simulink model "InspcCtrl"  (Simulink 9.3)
settings: Solver=FixedStepDiscrete  StartTime=0.0  StopTime=100000  FixedStep=Tstep  RelTol=1e-3  EnableMultiTasking=on
PreLoadFcn:
  | InspcCtrl.InspcCtrl_init();
InitFcn:
  | InspcCtrl.InspcCtrl_init();
StartFcn:
  | InspcCtrl.InspcCtrl_init();
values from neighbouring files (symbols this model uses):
  Tinit = 0.001    [InspcCtrl_init.m]    (also in TestOrthOscObjO_init.m = 0.1; TestOrthOsc_init.m; Test_PIDctrl_init.m; Test_LibVishia_Inspc_init.m = 0.002)
  Tstep = 0.0001    [InspcCtrl_init.m]    (also in TestOrthOscObjO_init.m = 0.0005; stimuli_Smlk.m = 0.001; TestOrthOsc_init.m = 5e-05; Test_PIDctrl_init.m)
undefined symbols (not defined in the file or in its folder): intmax, s1, s2, T1, test, TIs, v2, validy
libraries: libVishia_Inspc x36, libVishia_Ctrl x3, libVishia_CtrlSfn x2, libVishia_Conv x2, simulink x1

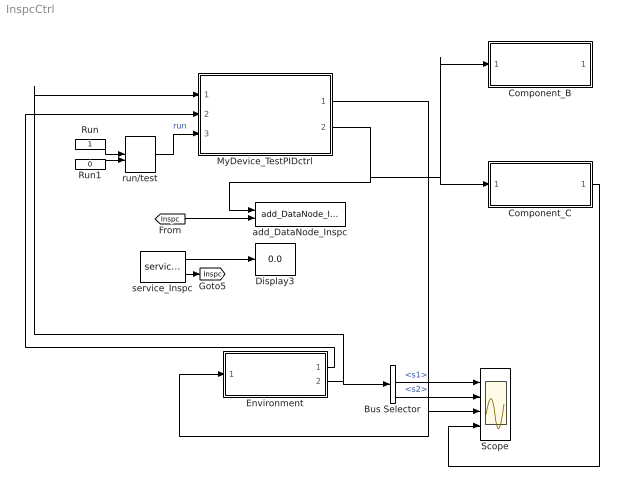
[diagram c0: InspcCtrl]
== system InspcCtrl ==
  Bus Selector : BusSelector  OutputSignals=s1,s2
  Component_B : Subsystem  Commented=on
  Component_C : Subsystem
  Display3 : Display
  Environment : Subsystem
  MyDevice_TestPIDctrl : Subsystem
  Run : Constant  OutDataTypeStr=boolean
  Run1 : Constant  Value=0  OutDataTypeStr=boolean
  Scope : Scope  NumInputPorts=4
  add_DataNode_Inspc : libVishia_Inspc/add_DataNode_Inspc  name1Refl='myDevice'  name2Refl=''
  run/test : ManualSwitch  CurrentSetting=0
  service_Inspc : libVishia_Inspc/service_Inspc  Tstep=Tstep  IpPort='UDP:0.0.0.0:60094'
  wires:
  MyDevice_TestPIDctrl/1(Out1) -> Environment/1(In1), Scope/3
  Environment/2(Out1) -> MyDevice_TestPIDctrl/1(In1), Bus Selector/1
  Bus Selector/1 -> Scope/1  "<s1>"
  service_Inspc/2 -> [Inspc]
  service_Inspc/1 -> Display3/1
  [Inspc] -> add_DataNode_Inspc/2
  MyDevice_TestPIDctrl/2(Out2) -> add_DataNode_Inspc/1, Component_B/1(In1), Component_C/1(In1)
  Bus Selector/2 -> Scope/2  "<s2>"
  Run/1 -> run/test/1
  Run1/1 -> run/test/2
  run/test/1 -> MyDevice_TestPIDctrl/3(In2)  "run"
  Environment/1(Out2) -> MyDevice_TestPIDctrl/2(In3)
  Component_C/1(Out1) -> Scope/4

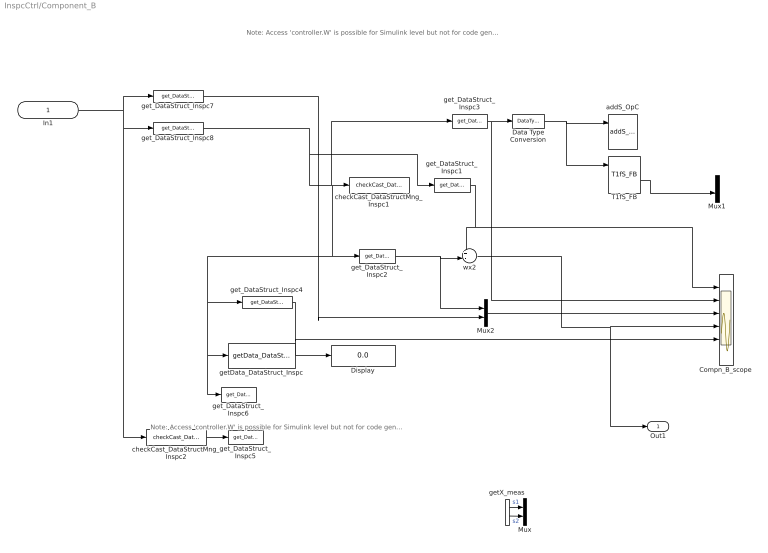
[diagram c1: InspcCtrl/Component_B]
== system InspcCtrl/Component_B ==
  note: Note: Access 'controller.W' is possible for Simulink level but not for code generation. Necessary to create special parameter in runtime. The necessary information for code generation are available only after init_... war run. With String processing in tlc it may be able. But tlc as less features for String processing.
  note: Note: Access 'controller.W' is possible for Simulink level but not for code generation. Necessary to create special parameter in runtime. The necessary information for code generation are available only after init_... war run. With String processing in tlc it may be able. But tlc as less features for String processing.
  In1 : Inport  OutDataTypeStr=uint32  PortDimensions=1  SampleTime=Tinit
  Compn_B_scope : Scope  NumInputPorts=6
  Data Type Conversion : DataTypeConversion  OutDataTypeStr=double
  Display : Display
  Mux : Mux  Commented=on  Inputs=2
  Mux1 : Mux  Inputs=2
  Mux2 : Mux  Inputs=2
  T1fS_FB : libVishia_Ctrl/T1fS_FB  T1=100  P_TA=Tstep
  addS_OpC : libVishia_Ctrl/addS_OpC  init=0  Tstep=-1
  checkCast_DataStructMng_Inspc1 : libVishia_Inspc/checkCast_DataStruct_Inspc  Commented=on  typeData='Controller_B_ObjMod'  headerfile=''
  checkCast_DataStructMng_Inspc2 : libVishia_Inspc/checkCast_DataStruct_Inspc  Commented=on  typeData='Device_ObjMod'  headerfile=''
  getData_DataStruct_Inspc : libVishia_Inspc/getData_DataStruct_Inspc  Commented=on  Tstep=Tstep  show='wxP'  typeName='F: wxP'  typedata=''  datapath='pid2'  header=''
  getX_meas : S-Function  Commented=on  FunctionName=out_MeasPrep_ProgrSimpleExmplA_SfOp  SFunctionDeploymentMode=off  EnableBusSupport=off
  get_DataStruct_Inspc1 : libVishia_Inspc/get_DataStruct_Inspc  show='test'  Tstep=Tstep  name1='F2:test'  headerfile=''
  get_DataStruct_Inspc2 : libVishia_Inspc/get_DataStruct_Inspc  show='xs'  Tstep=Tstep  name1='F2:xs'  headerfile=''
  get_DataStruct_Inspc3 : libVishia_Inspc/get_DataStruct_Inspc  show='yctrl'  Tstep=Tstep  name1='F2:yctrl'  headerfile=''
  get_DataStruct_Inspc4 : libVishia_Inspc/get_DataStruct_Inspc  show='controller.W'  Tstep=Tstep  name1="'F:  pid2.wxP'"  headerfile=''
  get_DataStruct_Inspc5 : libVishia_Inspc/get_DataStruct_Inspc  Commented=on  show='show'  Tstep=Tstep  name1='W'  headerfile=''
  get_DataStruct_Inspc6 : libVishia_Inspc/get_DataStruct_Inspc  Commented=on  show='s'  Tstep=Tstep  name1='s'  headerfile=''
  get_DataStruct_Inspc7 : libVishia_Inspc/get_DataStruct_Inspc  show='controller.W'  Tstep=Tstep  name1="'(Device_ObjMod*) F2:  controller.W'"  headerfile=''
  get_DataStruct_Inspc8 : libVishia_Inspc/get_DataStruct_Inspc  show='controller'  Tstep=Tinit  name1="'(Device_ObjMod*) Controller_ObjMod:  controller'"  headerfile=''
  wx2 : Sum  Inputs=+-|
  Out1 : Outport
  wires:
  In1/1 -> get_DataStruct_Inspc7/1, get_DataStruct_Inspc8/1, checkCast_DataStructMng_Inspc2/1
  get_DataStruct_Inspc1/1 -> wx2/1, Compn_B_scope/1
  Data Type Conversion/1 -> T1fS_FB/1, addS_OpC/1
  T1fS_FB/2 -> Mux1/2
  get_DataStruct_Inspc2/1 -> Mux2/1, wx2/2
  wx2/1 -> Out1/1, Compn_B_scope/4
  get_DataStruct_Inspc3/1 -> Compn_B_scope/2, Data Type Conversion/1
  get_DataStruct_Inspc8/1 -> get_DataStruct_Inspc1/1, checkCast_DataStructMng_Inspc1/1, get_DataStruct_Inspc4/1, getData_DataStruct_Inspc/1, get_DataStruct_Inspc6/1, get_DataStruct_Inspc2/1, get_DataStruct_Inspc3/1
  checkCast_DataStructMng_Inspc2/1 -> get_DataStruct_Inspc5/1
  get_DataStruct_Inspc4/1 -> Compn_B_scope/5, Display/1
  getX_meas/1 -> Mux/1  "s1"
  getX_meas/2 -> Mux/2  "s2"
  Mux/1 -> ?
  Mux2/1 -> Compn_B_scope/3
  get_DataStruct_Inspc7/1 -> Mux2/2

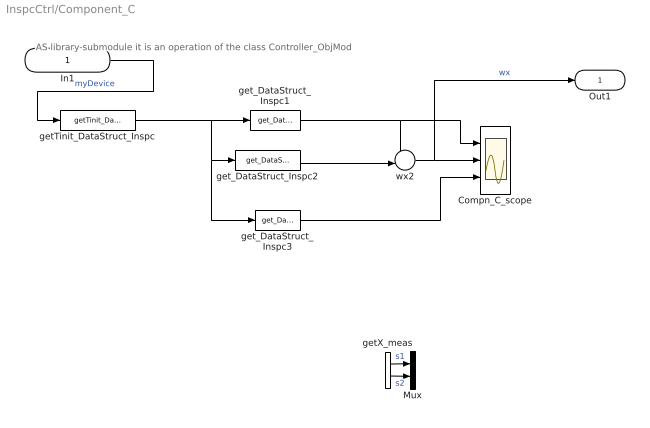
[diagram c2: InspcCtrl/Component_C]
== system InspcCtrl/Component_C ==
  note: AS library-submodule it is an operation of the class Controller_ObjMod
  In1 : Inport  OutDataTypeStr=uint32  PortDimensions=1  SampleTime=Tinit
  Compn_C_scope : Scope  NumInputPorts=3
  Mux : Mux  Commented=on  Inputs=2
  getTinit_DataStruct_Inspc : libVishia_Inspc/getTinit_DataStruct_Inspc  show='=controller'  typeName='(Device_ObjMod) controller: Controller_ObjMod '  headerfile='genSrcInspc/Controller_ObjMod.h'
  getX_meas : S-Function  Commented=on  FunctionName=out_MeasPrep_ProgrSimpleExmplA_SfOp  SFunctionDeploymentMode=off  EnableBusSupport=off
  get_DataStruct_Inspc1 : libVishia_Inspc/get_DataStruct_Inspc  show='W'  Tstep=Tstep  name1='W: F*2'  headerfile=''
  get_DataStruct_Inspc2 : libVishia_Inspc/get_DataStruct_Inspc  show='xs'  Tstep=Tstep  name1='xs: F*2'  headerfile=''
  get_DataStruct_Inspc3 : libVishia_Inspc/get_DataStruct_Inspc  show='yctrl'  Tstep=Tstep  name1='yctrl :F*2'  headerfile=''
  wx2 : Sum  Inputs=+-|
  Out1 : Outport
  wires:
  get_DataStruct_Inspc2/1 -> wx2/2
  getX_meas/1 -> Mux/1  "s1"
  getX_meas/2 -> Mux/2  "s2"
  wx2/1 -> Compn_C_scope/2, Out1/1  "wx"
  get_DataStruct_Inspc3/1 -> Compn_C_scope/3
  getTinit_DataStruct_Inspc/1 -> get_DataStruct_Inspc3/1, get_DataStruct_Inspc2/1, get_DataStruct_Inspc1/1
  In1/1 -> getTinit_DataStruct_Inspc/1  "myDevice"
  get_DataStruct_Inspc1/1 -> wx2/1, Compn_C_scope/1

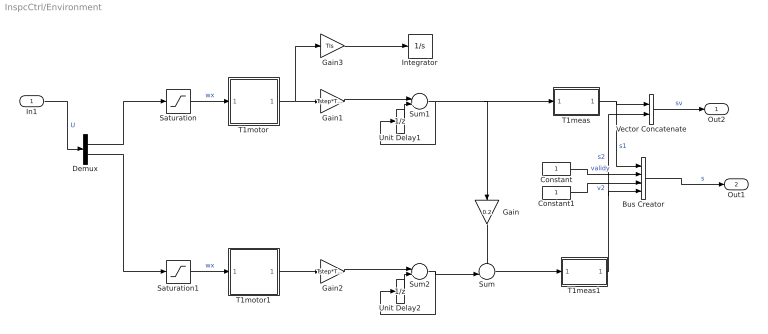
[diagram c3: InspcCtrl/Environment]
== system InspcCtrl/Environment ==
  In1 : Inport  PortDimensions=2
  Bus Creator : BusCreator  Inputs=s1,validy,v2,s2  OutDataTypeStr=Bus: Input_MeasPrep_ProgrSimpleExmplA
  Constant : Constant  OutDataTypeStr=uint16
  Constant1 : Constant  OutDataTypeStr=uint16
  Demux : Demux  Outputs=2
  Gain : Gain  Gain=0.2
  Gain1 : Gain  Gain=Tstep*TIs
  Gain2 : Gain  Gain=Tstep*TIs
  Gain3 : Gain  Commented=on  Gain=TIs
  Integrator : Integrator  Commented=on
  Saturation : Saturate
  Saturation1 : Saturate
  Sum : Sum  Inputs=++|
  Sum1 : Sum  Inputs=|++
  Sum2 : Sum  Inputs=|++
  T1meas : Subsystem
  T1meas1 : Subsystem
  T1motor : Subsystem
  T1motor1 : Subsystem
  Unit Delay1 : UnitDelay  SampleTime=-1  HasFrameUpgradeWarning=on
  Unit Delay2 : UnitDelay  SampleTime=-1  HasFrameUpgradeWarning=on
  Vector Concatenate : Concatenate
  Out2 : Outport  OutDataTypeStr=single
  Out1 : Outport  Port=2  OutDataTypeStr=Bus: Input_MeasPrep_ProgrSimpleExmplA
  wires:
  In1/1 -> Demux/1  "U"
  Saturation/1 -> T1motor/1(In2)  "wx"
  Gain1/1 -> Sum1/1
  T1motor/1(Out2) -> Gain3/1, Gain1/1
  Sum1/1 -> Gain/1, T1meas/1(In2), Unit Delay1/1
  Unit Delay1/1 -> Sum1/2
  Bus Creator/1 -> Out1/1  "s"
  T1meas/1(Out2) -> Vector Concatenate/1, Bus Creator/1  "s1"
  Demux/1 -> Saturation/1
  Demux/2 -> Saturation1/1
  Unit Delay2/1 -> Sum2/2
  T1motor1/1(Out2) -> Gain2/1
  Gain2/1 -> Sum2/1
  Saturation1/1 -> T1motor1/1(In2)  "wx"
  Sum2/1 -> Sum/2, Unit Delay2/1
  Sum/1 -> T1meas1/1(In2)
  Gain/1 -> Sum/1
  T1meas1/1(Out2) -> Vector Concatenate/2, Bus Creator/4  "s2"
  Gain3/1 -> Integrator/1
  Vector Concatenate/1 -> Out2/1  "sv"
  Constant/1 -> Bus Creator/2  "validy"
  Constant1/1 -> Bus Creator/3  "v2"

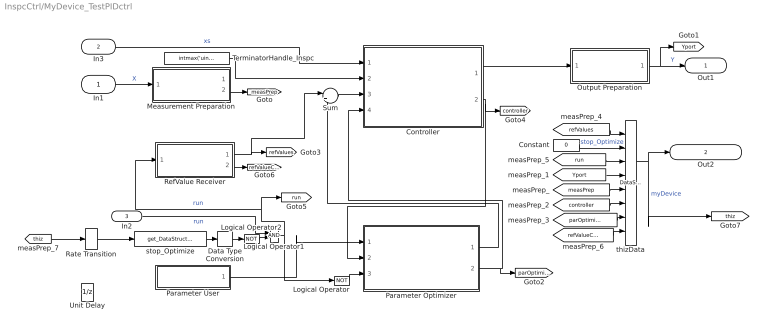
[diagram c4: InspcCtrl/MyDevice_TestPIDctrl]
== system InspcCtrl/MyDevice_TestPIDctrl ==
  In1 : Inport  OutDataTypeStr=Bus: Input_MeasPrep_ProgrSimpleExmplA
  In3 : Inport  Port=2  OutDataTypeStr=single  SampleTime=Tstep
  In2 : Inport  Port=3  OutDataTypeStr=boolean
  Constant : Constant  Value=0  OutDataTypeStr=uint16
  Controller : Subsystem
  Data Type Conversion : DataTypeConversion  OutDataTypeStr=boolean
  Logical Operator : Logic  Operator=NOT  IconShape=distinctive  AllPortsSameDT=off  OutDataTypeStr=boolean
  Logical Operator1 : Logic  IconShape=distinctive  AllPortsSameDT=off  OutDataTypeStr=boolean
  Logical Operator2 : Logic  Operator=NOT  IconShape=distinctive  AllPortsSameDT=off  OutDataTypeStr=boolean
  Measurement Preparation : Subsystem  Commented=on
  Output Preparation : Subsystem
  Parameter Optimizer : Subsystem
  Parameter User : Subsystem
  Rate Transition : RateTransition  OutPortSampleTime=Tstep
  RefValue Receiver : Subsystem
  Sum : Sum  Inputs=|++
  TerminatorHandle_Inspc : Constant  Value=intmax('uint32')  OutDataTypeStr=uint32  SampleTime=Tinit
  Unit Delay : UnitDelay  SampleTime=-1  HasFrameUpgradeWarning=on
  stop_Optimize : libVishia_Inspc/get_DataStruct_Inspc  show='stop_Optimize'  Tstep=Tstep  name1='(Device_ObjMod) stop_Optimize :W'  headerfile=''
  thizData : libVishia_Inspc/DataStructMng_Inspc  dirGenSource=dstPathGenDataStruct  typeData='Device_ObjMod'  inherit=off  chain=off  inputs=|
      | refValues;
      | =stop_Optimize;
      | run;
      | Yport;
      | measPrep :MeasPrep_ProgrSimpleExmplA ;
      | =controller :Controller_ObjMod;
      | =parOptimizer : ParamOptimizer_ObjMod;
      | =refValueCtrl :RefValueCtrl;
  Out1 : Outport  OutDataTypeStr=single  PortDimensions=2
  Out2 : Outport  Port=2  OutDataTypeStr=uint32  PortDimensions=1
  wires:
  RefValue Receiver/1(Out2) -> Sum/1, [refValues]
  Output Preparation/1(Out2) -> [Yport], Out1/1  "Y"
  Controller/1(Out2) -> Output Preparation/1(In3)
  Parameter Optimizer/1(Out1) -> Sum/2
  In1/1 -> Measurement Preparation/1(In1)  "X"
  Parameter User/1(Out2) -> Parameter Optimizer/1(In2)
  Logical Operator/1 -> Parameter Optimizer/3(In1)
  Logical Operator1/1 -> [run], RefValue Receiver/1(In1), Logical Operator/1  "run"
  Sum/1 -> Controller/3(In2)
  In3/1 -> Controller/1(In3)  "xs"
  [Yport] -> thizData/4
  [refValues] -> thizData/1
  Controller/2(Out3) -> Parameter Optimizer/2(In3), [controller]
  Measurement Preparation/2(Out2) -> [measPrep]
  thizData/1 -> [thiz], Out2/1  "myDevice"
  Parameter Optimizer/2(Out3) -> Controller/4(In4), [parOptimizer]
  [run] -> thizData/3
  [measPrep] -> thizData/5
  [controller] -> thizData/6
  [parOptimizer] -> thizData/7
  Constant/1 -> thizData/2  "stop_Optimize"
  RefValue Receiver/2(Out3) -> [refValueCtrl]
  [refValueCtrl] -> thizData/8
  TerminatorHandle_Inspc/1 -> Controller/2(In1)
  In2/1 -> Logical Operator1/1  "run"
  [thiz] -> Rate Transition/1
  Logical Operator2/1 -> Logical Operator1/2
  Data Type Conversion/1 -> Logical Operator2/1
  stop_Optimize/1 -> Data Type Conversion/1
  Rate Transition/1 -> stop_Optimize/1

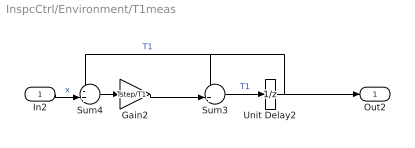
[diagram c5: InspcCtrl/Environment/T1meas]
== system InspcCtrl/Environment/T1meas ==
  In2 : Inport
  Gain2 : Gain  Gain=Tstep/T1
  Sum3 : Sum  Inputs=++|
  Sum4 : Sum  Inputs=-+|
  Unit Delay2 : UnitDelay  SampleTime=-1  HasFrameUpgradeWarning=on
  Out2 : Outport
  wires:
  Sum4/1 -> Gain2/1
  In2/1 -> Sum4/2  "x"
  Sum3/1 -> Unit Delay2/1  "T1"
  Gain2/1 -> Sum3/2
  Unit Delay2/1 -> Sum4/1, Sum3/1, Out2/1  "T1"

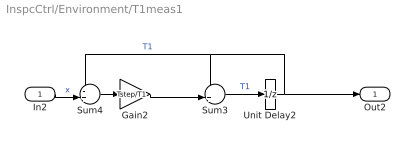
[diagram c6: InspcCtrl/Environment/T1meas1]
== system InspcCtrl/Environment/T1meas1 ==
  In2 : Inport
  Gain2 : Gain  Gain=Tstep/T1
  Sum3 : Sum  Inputs=++|
  Sum4 : Sum  Inputs=-+|
  Unit Delay2 : UnitDelay  SampleTime=-1  HasFrameUpgradeWarning=on
  Out2 : Outport
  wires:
  Sum4/1 -> Gain2/1
  In2/1 -> Sum4/2  "x"
  Sum3/1 -> Unit Delay2/1  "T1"
  Gain2/1 -> Sum3/2
  Unit Delay2/1 -> Sum4/1, Sum3/1, Out2/1  "T1"

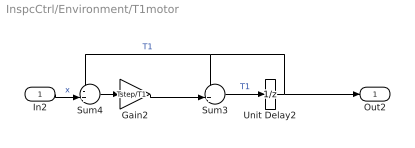
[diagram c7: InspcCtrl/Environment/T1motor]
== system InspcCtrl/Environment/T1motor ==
  In2 : Inport
  Gain2 : Gain  Gain=Tstep/T1
  Sum3 : Sum  Inputs=++|
  Sum4 : Sum  Inputs=-+|
  Unit Delay2 : UnitDelay  SampleTime=-1  HasFrameUpgradeWarning=on
  Out2 : Outport
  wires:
  Sum4/1 -> Gain2/1
  In2/1 -> Sum4/2  "x"
  Sum3/1 -> Unit Delay2/1  "T1"
  Gain2/1 -> Sum3/2
  Unit Delay2/1 -> Sum4/1, Sum3/1, Out2/1  "T1"

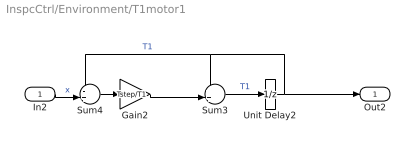
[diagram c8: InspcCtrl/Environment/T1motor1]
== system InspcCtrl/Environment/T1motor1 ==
  In2 : Inport
  Gain2 : Gain  Gain=Tstep/T1
  Sum3 : Sum  Inputs=++|
  Sum4 : Sum  Inputs=-+|
  Unit Delay2 : UnitDelay  SampleTime=-1  HasFrameUpgradeWarning=on
  Out2 : Outport
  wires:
  Sum4/1 -> Gain2/1
  In2/1 -> Sum4/2  "x"
  Sum3/1 -> Unit Delay2/1  "T1"
  Gain2/1 -> Sum3/2
  Unit Delay2/1 -> Sum4/1, Sum3/1, Out2/1  "T1"

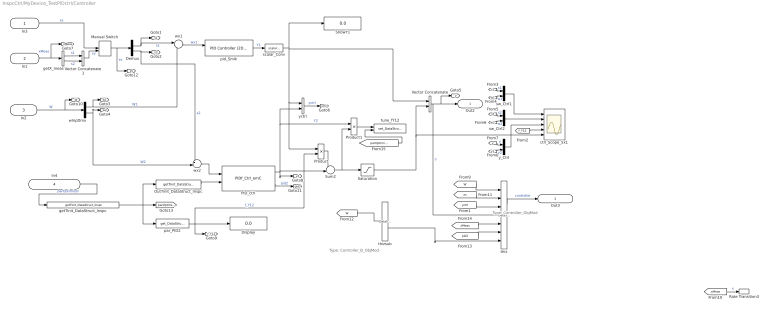
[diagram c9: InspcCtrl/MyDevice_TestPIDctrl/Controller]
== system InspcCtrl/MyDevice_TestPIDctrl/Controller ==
  note: Type: Controller_B_ObjMod
  note: Type: Controller_ObjMod
  In3 : Inport  OutDataTypeStr=single  PortDimensions=2  SampleTime=Tstep
  In1 : Inport  Port=2  OutDataTypeStr=uint32  PortDimensions=1  SampleTime=Tstep
  In2 : Inport  Port=3  OutDataTypeStr=single  PortDimensions=2  SampleTime=Tstep
  In4 : Inport  Port=4  OutDataTypeStr=uint32  PortDimensions=1  SampleTime=Tinit
  Demux : Demux  Outputs=2
  Display : Display
  Manual Switch : ManualSwitch
  OutTinit_DataStruct_Inspc : libVishia_Inspc/getTinit_DataStruct_Inspc  show='par_PID'  typeName='par_PID'  headerfile=''
  PID_ctrl : libVishia_CtrlSfn/PIDf_Ctrl_emC  Tstep=Tstep
  Product : Product
  Product1 : Product
  Rate Transition3 : RateTransition  Commented=on  OutPortSampleTime=Tinit
  Saturation : Saturate  UpperLimit=1  LowerLimit=-1
  ShowY1 : Display
  Sum2 : Sum  Inputs=++|
  Vector Concatenate : Concatenate
  Vector Concatenate1 : Concatenate
  ctrl_Scope_5x1 : Scope  NumInputPorts=5
  getTinit_DataStruct_Inspc : libVishia_Inspc/getTinit_DataStruct_Inspc  show='ParamOptimizer_ObjMod*'  typeName='(ParamOptimizer_ObjMod)'  headerfile=''
  getX_meas : S-Function  Commented=on  FunctionName=out_MeasPrep_ProgrSimpleExmplA_SfOp  SFunctionDeploymentMode=off  EnableBusSupport=off
  par_PID2 : libVishia_Inspc/get_DataStruct_Inspc  show='f_Y12'  Tstep=Tstep  name1='f_Y12 :F'  headerfile=''
  pid_Smlk : simulink/Continuous/PID Controller (2DOF)  Controller=PID  Form=Ideal  TimeDomain=Discrete-time  SampleTime=-1  IntegratorMethod=Backward Euler  FilterMethod=Forward Euler  ControllerParametersSource=internal  P=10  I=5  D=0  UseFilter=on  N=10  b=1  c=1  TunerSelectOption=Transfer Function Based (PID Tuner App)  InitialConditionSource=internal  InitialConditionForIntegrator=0  InitialConditionForFilter=0  DifferentiatorICPrevScaledInput=0  ExternalReset=none  TrackingMode=off  Kt=1  LimitOutput=on  UpperSaturationLimit=1.0  LowerSaturationLimit=-1.0  LinearizeAsGain=off  AntiWindupMode=back-calculation  Kb=1  POutMin=[]  POutMax=[]  IOutMin=[]  IOutMax=[]  DOutMin=[]  DOutMax=[]  NOutMin=[]  NOutMax=[]  bOutMin=[]  bOutMax=[]  cOutMin=[]  cOutMax=[]  SumOutMin=[]  SumOutMax=[]  SaturationOutMin=[]  SaturationOutMax=[]  PParamMin=[]  PParamMax=[]  IParamMin=[]  IParamMax=[]  DParamMin=[]  DParamMax=[]  NParamMin=[]  NParamMax=[]  bParamMin=[]  bParamMax=[]  cParamMin=[]  cParamMax=[]  KbParamMin=[]  KbParamMax=[]  KtParamMin=[]  KtParamMax=[]  KbOutMin=[]  KbOutMax=[]  KtOutMin=[]  KtOutMax=[]  IntegratorOutMin=[]  IntegratorOutMax=[]  FilterOutMin=[]  FilterOutMax=[]  SumI1OutMin=[]  SumI1OutMax=[]  SumI2OutMin=[]  SumI2OutMax=[]  SumI3OutMin=[]  SumI3OutMax=[]  SumI4OutMin=[]  SumI4OutMax=[]  SumDOutMin=[]  SumDOutMax=[]  Sum1OutMin=[]  Sum1OutMax=[]  Sum2OutMin=[]  Sum2OutMax=[]  Sum3OutMin=[]  Sum3OutMax=[]  DifferentiatorOutMin=[]  DifferentiatorOutMax=[]  FilterDiffOutCoefMin=[]  FilterDiffOutCoefMax=[]  ReciprocalOutMin=[]  ReciprocalOutMax=[]  SumDenOutMin=[]  SumDenOutMax=[]  SumNumOutMin=[]  SumNumOutMax=[]  DivideOutMin=[]  DivideOutMax=[]  IntegratorContinuousStateAttributes=''  IntegratorStateMustResolveToSignalObject=off  IntegratorRTWStateStorageClass=Auto  FilterContinuousStateAttributes=''  FilterStateMustResolveToSignalObject=off  FilterRTWStateStorageClass=Auto  ParallelPVariant=Passthrough  IdealPVariant=InternalParameters  IVariant=InternalParameters  DVariant=InternalParameters  bVariant=InternalParameters  cVariant=InternalParameters  IntegratorVariant=Discrete  SatVariant=Enabled  AWVariant=BackCalculation  PCopyVariant=Disabled  TRVariant=Disabled  FdbkBlocksVariant=Feedback  IdealPFdbkVariant=InternalParameters  SatFdbkVariant=Enabled  DerivativeFilterVariant=ForwardEulerFilter  NVariant=InternalParameters  NCopyVariant=Disabled  FilterICVariant=InternalICsFilter  IntegratorICVariant=InternalICs  ExternalResetVariant=Disabled  TRSumVariant=Passthrough  SumFdbkVariant=Enabled  SumVariant=Sum_PID
  scalar_Conv : libVishia_Conv/scalar_Conv  SystemSampleTime=-1
  sw_Ctrl1 : Mux  Inputs=2
  sw_Ctrl2 : Mux  Inputs=2
  thiz : libVishia_Inspc/DataStructMng_Inspc  dirGenSource=dstPathGenDataStruct  typeData='Controller_ObjMod'  inherit=on  chain=off  inputs=|
      | W;
      | xs; //
      | yctrl;
      | Y;
      | =xMeas :MeasPrep_ProgrSimpleExmplA -22;
      | =pid2 : PIDf_Ctrl_emC -22;
  thizsub : libVishia_Inspc/DataStructMng_Inspc  dirGenSource=dstPathGenDataStruct  typeData='Controller_B_ObjMod'  inherit=off  chain=off  inputs=test;
  tune_fY12 : libVishia_Inspc/set_DataStruct_Inspc  show='tune_fY12'  Tstep=Tstep  typeName='(ParamOptimizer_ObjMod) tune_fY12 :F'  headerfile=''
  wInpDmx : Demux  Outputs=2
  wx1 : Sum  Inputs=|-+
  wx2 : Sum  Inputs=-+|
  y_Ctrl : Mux  Inputs=2
  yctrl : Concatenate
  Out2 : Outport  OutDataTypeStr=single  SampleTime=Tstep
  Out3 : Outport  Port=2  OutDataTypeStr=uint32  PortDimensions=1  SampleTime=Tinit
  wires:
  In1/1 -> [xMeas], getX_meas/1  "xMeas"
  pid_Smlk/1 -> scalar_Conv/1  "Y1"
  wInpDmx/1 -> [w1], wx1/2  "W1"
  Demux/2 -> [s2], wx2/1  "s2"
  wx2/1 -> PID_ctrl/1
  Vector Concatenate/1 -> thiz/4, Out2/1, [y]  "Y"
  PID_ctrl/1 -> [y2], Sum2/2, Product1/1, yctrl/2  "Y2"
  sw_Ctrl2/1 -> ctrl_Scope_5x1/2
  PID_ctrl/3 -> [pid2]  "pid2"
  wx1/1 -> pid_Smlk/1  "wx1"
  Demux/1 -> [s1], wx1/1  "s1"
  sw_Ctrl1/1 -> ctrl_Scope_5x1/1
  wInpDmx/2 -> [w2], wx2/2  "W2"
  y_Ctrl/1 -> ctrl_Scope_5x1/3
  Sum2/1 -> Saturation/1, Product1/2
  Product/1 -> Sum2/1
  In2/1 -> [W], wInpDmx/1  "W"
  yctrl/1 -> [yctrl]  "yctrl"
  par_PID2/1 -> Display/1, [f_Y12], Product/2  "f_Y12"
  [s1] -> sw_Ctrl1/1  "s1"
  [w1] -> sw_Ctrl1/2  "w1"
  [w2] -> sw_Ctrl2/2  "w2"
  [s2] -> sw_Ctrl2/1  "s2"
  [y2] -> y_Ctrl/2  "y2"
  [y] -> y_Ctrl/1  "y"
  [xMeas] -> Rate Transition3/1  "x"
  In4/1 -> getTinit_DataStruct_Inspc/1  "parOptimizer"
  [yctrl] -> thiz/3
  [f_Y12] -> ctrl_Scope_5x1/4
  Saturation/1 -> ctrl_Scope_5x1/5, Vector Concatenate/2
  OutTinit_DataStruct_Inspc/1 -> PID_ctrl/2
  Product1/1 -> tune_fY12/1
  [W] -> thiz/1
  thiz/1 -> Out3/1  "controller"
  [W] -> thizsub/1
  [pid2] -> thiz/6
  scalar_Conv/1 -> ShowY1/1, Product/1, yctrl/1, Vector Concatenate/1
  Manual Switch/1 -> [xs], Demux/1  "xs"
  [xs] -> thiz/2
  thizsub/2 -> thiz/7
  getX_meas/1 -> Vector Concatenate1/1  "s1"
  getX_meas/2 -> Vector Concatenate1/2  "s2"
  In3/1 -> Manual Switch/1  "xs"
  Vector Concatenate1/1 -> Manual Switch/2  "sv"
  [xMeas] -> thiz/5
  [parOptimizer] -> tune_fY12/2
  getTinit_DataStruct_Inspc/1 -> par_PID2/1, [parOptimizer], OutTinit_DataStruct_Inspc/1

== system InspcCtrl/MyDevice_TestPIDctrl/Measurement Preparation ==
  In1 : Inport  OutDataTypeStr=Bus: Input_MeasPrep_ProgrSimpleExmplA
  S-Function : S-Function  FunctionName=step_MeasPrep_ProgrSimpleExmplA_SfH  Parameters=Tstep  SFunctionDeploymentMode=off  EnableBusSupport=off
  Out1 : Outport  OutDataTypeStr=uint32
  Out2 : Outport  Port=2  OutDataTypeStr=uint32
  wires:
  In1/1 -> S-Function/1  "X"
  S-Function/2 -> Out2/1  "MeasPrep"
  S-Function/1 -> Out1/1  "Xi"

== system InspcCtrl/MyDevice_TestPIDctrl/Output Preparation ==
  In3 : Inport
  Gain : Gain
  Out2 : Outport
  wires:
  Gain/1 -> Out2/1  "Yport"
  In3/1 -> Gain/1  "Yi"

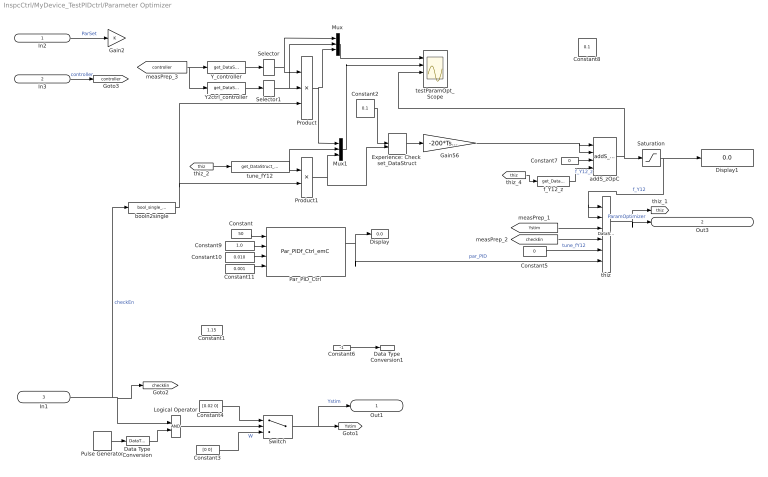
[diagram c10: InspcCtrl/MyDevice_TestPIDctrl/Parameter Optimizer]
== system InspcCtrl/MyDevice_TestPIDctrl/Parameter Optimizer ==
  In2 : Inport  OutDataTypeStr=uint32  PortDimensions=1  SampleTime=Tinit
  In3 : Inport  Port=2  OutDataTypeStr=uint32  PortDimensions=1  SampleTime=Tinit
  In1 : Inport  Port=3  OutDataTypeStr=boolean  PortDimensions=1
  Constant : Constant  Value=50  OutDataTypeStr=single  SampleTime=-1
  Constant1 : Constant  Value=1.15  OutDataTypeStr=single
  Constant10 : Constant  Value=0.010  OutDataTypeStr=single  SampleTime=-1
  Constant11 : Constant  Value=0.001  OutDataTypeStr=single  SampleTime=-1
  Constant2 : Constant  Value=0.1  OutDataTypeStr=single
  Constant3 : Constant  Value=[0 0]  OutDataTypeStr=single
  Constant4 : Constant  Value=[0.02 0]  OutDataTypeStr=single
  Constant5 : Constant  Value=0  OutDataTypeStr=single
  Constant6 : Constant  Commented=on  Value=-1  OutDataTypeStr=int32
  Constant7 : Constant  Value=0  OutDataTypeStr=boolean
  Constant8 : Constant  Commented=on  Value=0.1  OutDataTypeStr=single
  Constant9 : Constant  Value=1.0  OutDataTypeStr=single  SampleTime=-1
  Data Type Conversion : DataTypeConversion  OutDataTypeStr=boolean
  Data Type Conversion1 : DataTypeConversion  Commented=on  OutDataTypeStr=uint32
  Display : Display
  Display1 : Display
  Experience: Check  set_DataStruct : ManualSwitch  CurrentSetting=0
  Gain2 : Gain
  Gain56 : Gain  Gain=-200*Tstep
  Logical Operator : Logic  IconShape=distinctive  AllPortsSameDT=off  OutDataTypeStr=boolean
  Mux : Mux  Inputs=3
  Mux1 : Mux  Inputs=3
  Par_PID_Ctrl : libVishia_CtrlSfn/Par_PIDf_Ctrl_emC  Tparam=Tparam  Tctrl=0.001  yMax=1.2
  Product : Product  Inputs=3
  Product1 : Product
  Pulse Generator : DiscretePulseGenerator  Period=50000  PulseWidth=25000  SampleTime=Tstep
  Saturation : Saturate  UpperLimit=0  LowerLimit=-0.9
  Selector : Selector  IndexMode=Zero-based  InputPortWidth=2  IndexOptions=Index vector (dialog)  Indices=[1]  OutputSizes=1
  Selector1 : Selector  IndexMode=Zero-based  InputPortWidth=2  IndexOptions=Index vector (dialog)  Indices=[1]  OutputSizes=1
  Switch : Switch  Criteria=u2 ~= 0
  Y2ctrl_controller : libVishia_Inspc/get_DataStruct_Inspc  show='show'  Tstep=Tstep  name1='(Controller_ObjMod) yctrl:F*2'  headerfile=''
  Y_controller : libVishia_Inspc/get_DataStruct_Inspc  show='show'  Tstep=Tstep  name1='(Controller_ObjMod) Y:F*2'  headerfile=''
  addS_zOpC : libVishia_Ctrl/addS_zOpC
  booln2single : libVishia_Conv/bool_single_FB  hi=1.0  lo=0
  f_Y12_z : libVishia_Inspc/get_DataStruct_Inspc  show='f_Y12'  Tstep=Tstep  name1='f_Y12:F'  headerfile=''
  testParamOpt_Scope : Scope  NumInputPorts=4
  thiz : libVishia_Inspc/DataStructMng_Inspc  dirGenSource=dstPathGenDataStruct  typeData='ParamOptimizer_ObjMod'  inherit=off  chain=off  inputs=|
      | -9 f_Y12;
      | -44 reserve;
      | Ystim;
      | -9 checkEn;
      | -30=tune_fY12;
      | -11=par_PID :ParFactors_PIDf_Ctrl_emC ;
  tune_fY12 : libVishia_Inspc/get_DataStruct_Inspc  show='tune_fY12'  Tstep=Tstep  name1='tune_fY12 :F'  headerfile=''
  Out1 : Outport  OutDataTypeStr=single  PortDimensions=2
  Out3 : Outport  Port=2  OutDataTypeStr=uint32  PortDimensions=1  SampleTime=Tinit
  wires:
  Par_PID_Ctrl/1 -> Display/1, thiz/6  "par_PID"
  In2/1 -> Gain2/1  "ParSet"
  Switch/1 -> [Ystim], Out1/1  "Ystim"
  Constant1/1 -> ?
  Constant3/1 -> Switch/3  "W"
  Constant4/1 -> Switch/1
  Pulse Generator/1 -> Data Type Conversion/1
  Logical Operator/1 -> Switch/2
  Data Type Conversion/1 -> Logical Operator/2
  In1/1 -> booln2single/1, [checkEn], Logical Operator/1  "checkEn"
  Saturation/1 -> Display1/1, thiz/2, thiz/1  "f_Y12"
  Constant6/1 -> Data Type Conversion1/1
  thiz/1 -> Out3/1, [thiz]  "ParamOptimizer"
  [Ystim] -> thiz/3
  [checkEn] -> thiz/4
  In3/1 -> [controller]  "controller"
  [controller] -> Y_controller/1, Y2ctrl_controller/1
  Y_controller/1 -> Selector/1
  Y2ctrl_controller/1 -> Selector1/1
  Product/1 -> Mux1/1, Mux/3
  addS_zOpC/1 -> testParamOpt_Scope/3, Saturation/1
  Gain56/1 -> addS_zOpC/2, addS_zOpC/1
  [thiz] -> f_Y12_z/1
  f_Y12_z/1 -> addS_zOpC/4  "f_Y12_z"
  booln2single/1 -> Product1/2, Product/3
  Mux/1 -> testParamOpt_Scope/1
  Constant5/1 -> thiz/5  "tune_fY12"
  [thiz] -> tune_fY12/1
  tune_fY12/1 -> Product1/1, Mux1/2
  Experience: Check  set_DataStruct/1 -> Gain56/1
  Product1/1 -> Experience: Check  set_DataStruct/2, Mux1/3
  Mux1/1 -> testParamOpt_Scope/2
  Constant7/1 -> addS_zOpC/3
  Selector/1 -> Mux/1, Product/1
  Selector1/1 -> Mux/2, Product/2
  Constant/1 -> Par_PID_Ctrl/1
  Constant2/1 -> Experience: Check  set_DataStruct/1
  Constant9/1 -> Par_PID_Ctrl/2
  Constant10/1 -> Par_PID_Ctrl/3
  Constant11/1 -> Par_PID_Ctrl/4

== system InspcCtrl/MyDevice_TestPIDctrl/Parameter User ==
  Constant : Constant  OutDataTypeStr=uint32
  Out2 : Outport
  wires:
  Constant/1 -> Out2/1  "ParSet"

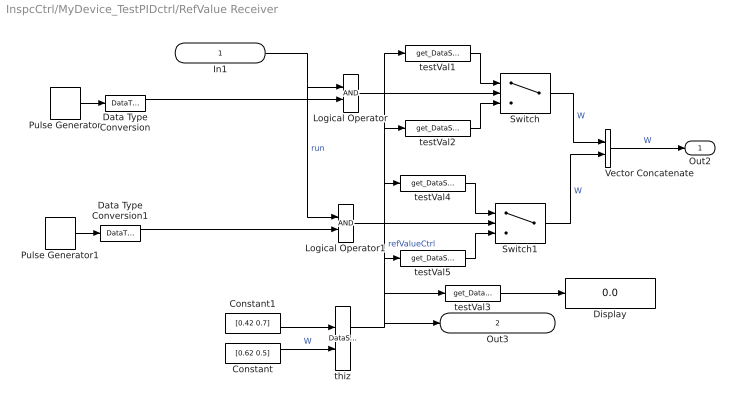
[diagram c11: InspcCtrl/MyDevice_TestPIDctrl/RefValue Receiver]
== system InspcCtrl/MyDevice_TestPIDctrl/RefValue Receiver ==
  In1 : Inport  OutDataTypeStr=boolean
  Constant : Constant  Value=[0.62 0.5]  OutDataTypeStr=single
  Constant1 : Constant  Value=[0.42 0.7]  OutDataTypeStr=single
  Data Type Conversion : DataTypeConversion  OutDataTypeStr=boolean
  Data Type Conversion1 : DataTypeConversion  OutDataTypeStr=boolean
  Display : Display
  Logical Operator : Logic  IconShape=distinctive  AllPortsSameDT=off  OutDataTypeStr=boolean
  Logical Operator1 : Logic  IconShape=distinctive  AllPortsSameDT=off  OutDataTypeStr=boolean
  Pulse Generator : DiscretePulseGenerator  Period=100000  PulseWidth=50000  SampleTime=Tstep
  Pulse Generator1 : DiscretePulseGenerator  Period=100000  PulseWidth=50000  PhaseDelay=25000  SampleTime=Tstep
  Switch : Switch  Criteria=u2 ~= 0
  Switch1 : Switch  Criteria=u2 ~= 0
  Vector Concatenate : Concatenate
  testVal1 : libVishia_Inspc/get_DataStruct_Inspc  show='testVal1[0]'  Tstep=Tstep  name1='testVal1[0] :F'  headerfile=''
  testVal2 : libVishia_Inspc/get_DataStruct_Inspc  show='testVal2[0]'  Tstep=Tstep  name1='testVal2[0] :F'  headerfile=''
  testVal3 : libVishia_Inspc/get_DataStruct_Inspc  show='testVal2'  Tstep=Tstep  name1='testVal2[1] :F'  headerfile=''
  testVal4 : libVishia_Inspc/get_DataStruct_Inspc  show='testVal1[1]'  Tstep=Tstep  name1='testVal1[1] :F'  headerfile=''
  testVal5 : libVishia_Inspc/get_DataStruct_Inspc  show='testVal2[1]'  Tstep=Tstep  name1='testVal2[1] :F'  headerfile=''
  thiz : libVishia_Inspc/DataStructMng_Inspc  dirGenSource=dstPathGenDataStruct  typeData='RefValueCtrl'  inherit=off  chain=off  inputs=|
      | =testVal1 :F*2;
      | =testVal2 :F*2;
  Out2 : Outport
  Out3 : Outport  Port=2  OutDataTypeStr=uint32  PortDimensions=1  SampleTime=Tinit
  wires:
  Vector Concatenate/1 -> Out2/1  "W"
  Pulse Generator/1 -> Data Type Conversion/1
  Data Type Conversion/1 -> Logical Operator/2
  Constant1/1 -> thiz/1
  Constant/1 -> thiz/2  "W"
  In1/1 -> Logical Operator1/1, Logical Operator/1  "run"
  Logical Operator/1 -> Switch/2
  testVal1/1 -> Switch/1
  testVal2/1 -> Switch/3
  thiz/1 -> Out3/1, testVal5/1, testVal4/1, testVal2/1, testVal1/1, testVal3/1  "refValueCtrl"
  testVal3/1 -> Display/1
  Data Type Conversion1/1 -> Logical Operator1/2
  Pulse Generator1/1 -> Data Type Conversion1/1
  Logical Operator1/1 -> Switch1/2
  testVal5/1 -> Switch1/3
  testVal4/1 -> Switch1/1
  Switch/1 -> Vector Concatenate/1  "W"
  Switch1/1 -> Vector Concatenate/2  "W"
